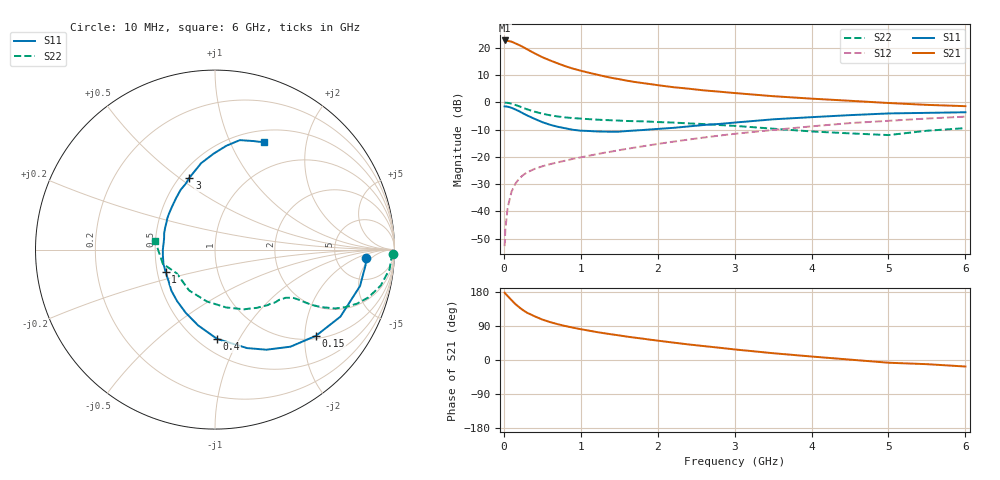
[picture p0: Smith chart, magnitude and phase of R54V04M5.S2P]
! SIEMENS Small Signal Semiconductors
! BFR183
! Si NPN RF Bipolar Junction Transistor in SOT23
! VCE = 4 V  IC = 4.5 mA
! Common Emitter S-Parameters:  May  1996
# GHz  S  MA  R  50
!  f  S11  S21  S12  S22
! GHz  MAG  ANG  MAG  ANG  MAG  ANG  MAG  ANG
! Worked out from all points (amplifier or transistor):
!   36 points, 10 MHz to 6 GHz, reference 50 ohm
!   highest |S21| = 22.7 dB at 10 MHz (marker M1)
!   |S21| within 3 dB of that: start of sweep to 287.1 MHz
!   unconditionally stable (mu >= 1): 1.11 GHz to 2.673 GHz
!   at 250 MHz: K = 0.40, MSG = 23.5 dB, |S12| = -26.7 dB
!   at 1.4 GHz: K = 1.06, MAG = 12.0 dB, |S12| = -18.1 dB
!   at 6 GHz: K = 0.88, MSG = 1.9 dB, |S12| = -5.3 dB
!   S11 on the Smith chart (normalised r, x): 10 MHz: 11, -3; 150 MHz: 1.07, -2.28; 400 MHz: 0.61, -0.81; 1 GHz: 0.55, -0.15; 3 GHz: 0.56, +0.55; 6 GHz: 0.64, +1.35
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0.01  0.8416 -3.0  13.63 177.8  0.0023 89.8  0.991 -1.3
0.02  0.8435 -5.8  13.57 175.2  0.0047 84.6  0.9841 -2.6
0.05  0.8331 -14.1  13.38 168.7  0.0118 82.4  0.9788 -6.4
0.1  0.7925 -28.1  12.97 158.0  0.023 76.6  0.9451 -12.2
0.15  0.7396 -40.5  12.05 147.6  0.0322 70.0  0.8955 -17.3
0.2  0.6853 -52.1  11.21 139.1  0.04 65.3  0.8456 -20.9
0.25  0.6272 -62.8  10.34 131.4  0.0463 61.2  0.7921 -23.9
0.3  0.5769 -72.0  9.426 124.9  0.0517 59.1  0.7458 -26.1
0.4  0.4974 -88.7  7.916 115.4  0.0601 55.9  0.6739 -28.4
0.5  0.4329 -102.5  6.722 106.7  0.0671 54.6  0.6188 -29.8
0.6  0.388 -114.9  5.874 100.1  0.0734 54.5  0.5788 -30.4
0.7  0.3564 -126.3  5.183 94.5  0.0792 54.5  0.5507 -30.8
0.8  0.3338 -136.8  4.597 89.6  0.0852 54.7  0.529 -31.2
1  0.3019 -155.8  3.796 81.3  0.0979 56.0  0.5028 -32.2
1.1  0.2983 -164.2  3.503 77.7  0.1045 56.6  0.4919 -33.1
1.6  0.2976 162.1  2.495 61.7  0.1402 58.1  0.4548 -37.9
2.2  0.3399 134.4  1.897 46.0  0.1895 56.9  0.4257 -46.8
3  0.4251 109.6  1.48 27.9  0.2646 51.3  0.3702 -64.0
3.5  0.4877 99.1  1.296 17.9  0.311 46.2  0.3285 -79.0
4.5  0.5824 83.7  1.067 1.0  0.4158 34.5  0.2694 -122.5
5.5  0.6409 70.7  0.898 -11.0  0.5045 21.8  0.301 -164.8
6  0.6568 65.6  0.85 -17.2  0.5462 13.7  0.3366 172.0
